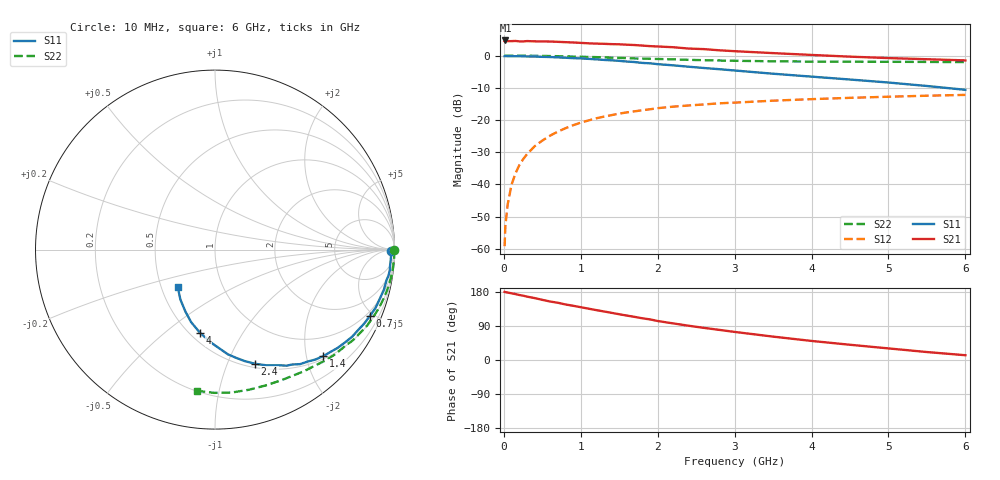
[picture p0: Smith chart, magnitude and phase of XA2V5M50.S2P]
! SIEMENS Discrete & RF Semiconductors
! BFY180
! Si NPN RF Bipolar Junction Transistor in MICRO-X
! VCE = 2.5 V  IC = 0.5 mA
! Common Emitter S-Parameters:  May  1997
# GHz  S  MA  R  50
!  f  S11  S21  S12  S22
! GHz  MAG  ANG  MAG  ANG  MAG  ANG  MAG  ANG
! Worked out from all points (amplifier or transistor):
!   36 points, 10 MHz to 6 GHz, reference 50 ohm
!   highest |S21| = 4.7 dB at 20 MHz (marker M1)
!   |S21| within 3 dB of that: start of sweep to 2.77 GHz
!   unconditionally stable (mu >= 1): 5.433 GHz to end of sweep
!   at 250 MHz: K = 0.06, MSG = 18.3 dB, |S12| = -32.2 dB
!   at 1.4 GHz: K = 0.40, MSG = 11.0 dB, |S12| = -18.5 dB
!   at 6 GHz: K = 1.02, MAG = 4.5 dB, |S12| = -12.2 dB
!   S11 on the Smith chart (normalised r, x): 10 MHz: open; 700 MHz: 0.76, -4.73; 1.4 GHz: 0.56, -2.32; 2.4 GHz: 0.54, -1.26; 4 GHz: 0.56, -0.67; 6 GHz: 0.61, -0.28
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0.01  0.9809 -0.3  1.669 179.9  0.0011 84.0  0.9988 -0.1
0.02  0.983 -0.9  1.72 179.0  0.0023 99.0  0.9999 -0.5
0.05  0.9813 -1.7  1.679 178.0  0.0049 83.1  0.9986 -1.1
0.1  0.9809 -3.3  1.679 176.0  0.0099 88.7  0.9992 -2.3
0.2  0.9807 -6.7  1.666 171.6  0.0198 84.8  0.9972 -4.6
0.3  0.9705 -10.1  1.682 167.3  0.0294 81.8  0.9953 -6.9
0.4  0.9673 -13.3  1.667 163.4  0.0391 80.1  0.993 -9.1
0.6  0.9518 -19.9  1.656 154.4  0.0571 74.7  0.9844 -13.6
0.7  0.9385 -23.3  1.638 151.1  0.0659 71.9  0.9794 -15.8
0.8  0.9278 -26.4  1.618 146.6  0.0745 69.5  0.9734 -18.0
1.1  0.8908 -35.4  1.553 135.5  0.0985 61.9  0.9535 -24.3
1.4  0.8458 -44.6  1.508 124.5  0.1192 55.4  0.93 -30.4
1.7  0.7949 -53.4  1.46 113.8  0.1365 49.4  0.903 -36.0
2.2  0.7067 -65.9  1.351 96.6  0.1613 40.4  0.8741 -44.6
2.4  0.6731 -70.8  1.288 90.5  0.1682 37.5  0.86 -47.6
2.6  0.6427 -75.1  1.262 84.8  0.1746 34.8  0.849 -50.5
3  0.5877 -83.0  1.172 74.1  0.1863 29.4  0.8312 -56.3
3.5  0.5236 -91.6  1.094 61.7  0.1998 24.1  0.8166 -62.9
4  0.4719 -100.1  1.025 50.3  0.211 18.8  0.8077 -69.6
4.5  0.4256 -108.2  0.964 40.2  0.2211 14.0  0.8035 -76.3
5.5  0.3377 -124.9  0.879 21.0  0.2385 4.9  0.7983 -90.2
6  0.2945 -134.8  0.843 12.6  0.2457 0.1  0.793 -97.2
